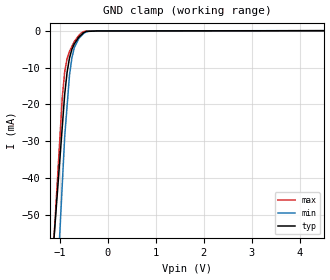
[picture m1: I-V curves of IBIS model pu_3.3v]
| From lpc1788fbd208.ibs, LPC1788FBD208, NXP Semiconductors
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[Model] pu_3.3v
Model_type Input
Vinl = 990.000mV
Vinh = 2.31000V
C_comp 900.000fF 855.000fF 945.000fF
| variable typ   min   max
[Voltage Range] 3.30000V 3.00000V 3.60000V
[POWER Clamp Reference] 3.30000V 3.00000V 3.60000V
[GND Clamp Reference] 0.00000V 0.00000V 0.00000V
[Temperature Range]   25   85   -40
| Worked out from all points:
|   GND clamp passes 1 mA (typ) near -0.54 V on its own axis
[GND Clamp]
-3.3V     -438.5mA   -646.2mA   -539.2mA
-950mV    -26.12mA   -41.76mA   -18.22mA
-900mV    -17.35mA   -28.9mA    -11.22mA
-850mV    -11.36mA   -20.52mA   -7.6mA
-800mV    -7.442mA   -12.15mA   -5.625mA
-750mV    -5.079mA   -7.409mA   -4.294mA
-700mV    -3.596mA   -4.64mA    -2.964mA
-600mV    -1.693mA   -2.032mA   -1.181mA
-500mV    -488.5uA   -682uA     -233.7uA
-400mV    -173.2uA   -129.9uA   -101.2uA
-200mV    -62.56uA   -47.1uA    -77.07uA
6.6V      35.04uA    32.39uA    35.06uA
[POWER Clamp]
-3.3V     0A         0A         0A
6.6V      0A         0A         0A
